| IBIS file stm32mp151_153xad_tfbga257.ibs
[IBIS ver]   4.2
[File name]   stm32mp151_153xad_tfbga257.ibs
[File Rev]   2.2
[Date]   07-07-2026
[Source]   Data Created at STMicroelectronics
[Disclaimer]  This information is for modeling purpose only and is
   not guaranted.
   The information is subject to change without notice.
[Copyright]   Copyright 2026 STMicroelectronics Inc.
|   Component stm32mp151_153xad_tfbga257
[Component] stm32mp151_153xad_tfbga257
[Manufacturer] STMicroelectronics
[Package]
| variable   typ   min   max
R_pkg  4.52E-01  1.78E-01  6.98E-01
L_pkg  2.44E-09  9.38E-10  4.05E-09
C_pkg  6.28E-13  3.36E-13  3.08E-12
[Pin]   signal_name   model_name
1A1  PE1  io8_ft
1A2  PD10  io8_ft_hslv
1A3  PE3  io8_ft_hslv
1A4  PB14  io8_ft_hslv
1A5  PD2  io8_ft_hslv
1A6  VSS  gnd
1A7  VDD1V2_Unused  nc
1A8  DDR_ZQ  nc
1A9  DDR_A7  PDDRIO_PAD
1B1  PD6  io8_ft_hslv
1B2  PE14  io8_ft_hslv
1B3  VDDCORE  power
1B4  PC12  io8_ft_hslv
1B5  VDDCORE  power
1B6  VDDA1V8_Unused  nc
1B7  VDD1V2_Unused  nc
1B8  VSS  gnd
1B9  VDDQ_DDR  power
1C1  PD9  io8_ft
1C2  PD15  io8_ft
1C3  VSS  gnd
1C4  VDDCORE  power
1C5  VSS  gnd
1C6  VDDCORE  power
1C7  VSS  gnd
1C8  DDR_DTO1  PDDRIO_PAD
1C9  DDR_A5  PDDRIO_PAD
1D1  VBAT  power
1D2  VSS  gnd
1D3  VDDCORE  power
1D4  VSS  gnd
1D5  VDDCORE  power
1D6  VSS  gnd
1D7  VDDCORE  power
1D8  DDR_DTO0  PDDRIO_PAD
1D9  VDDQ_DDR  power
1E1  PD14  io8_ft
1E2  VDD  power
1E3  VSS  gnd
1E4  VDDCORE  power
1E5  VSS  gnd
1E6  VDDCORE  power
1E7  VSS  gnd
1E8  VDDCORE  power
1E9  DDR_RASN  PDDRIO_PAD
1F1  VDDA  nc
1F2  VDDA  nc
1F3  VDD  power
1F4  VSS  gnd
1F5  VDDCORE  power
1F6  VSS  gnd
1F7  VDDCORE  power
1F8  DDR_ATO  nc
1F9  VDDQ_DDR  power
1G1  VSSA  gnd
1G2  VSS  gnd
1G3  VDD  power
1G4  VDD  power
1G5  VSS  gnd
1G6  VDDCORE  power
1G7  VSS  gnd
1G8  VDDCORE  power
1G9  DDR_A6  PDDRIO_PAD
1H1  PA5  io8_ft_hslv
1H2  VSS  gnd
1H3  VSS  gnd
1H4  VSS  gnd
1H5  VDDA1V8_REG  nc
1H6  VSS  gnd
1H7  VDD3V3_USB  power
1H8  VSS  gnd
1H9  VDDQ_DDR  power
1J1  PA4  io8_ft
1J2  PB13  io8_ft_hslv_et
1J3  VDD_OTP  power
1J4  PE9  io8_ft_hslv
1J5  VSS  gnd
1J6  VDDA1V1_REG  nc
1J7  PF10  io8_ft_hslv
1J8  USB_RREF  nc
1J9  VSS  gnd
A1  VSS  gnd
A2  PD1  io8_ft_hslv
A3  PB7  io8_ft_hslv
A4  PC6  io8_ft_hslv
A6  VSS  gnd
A7  PD3  io8_ft_hslv
A9  PC8  io8_ft_hslv
A10  PE4  io8_ft_hslv
A12  DNU  nc
A13  DNU  nc
A15  JTDO-TRACESWO  io8_ft
A16  JTCK-SWCLK  isudqf
A17  DDR_DQ0  PDDRIO_PAD
A18  DDR_DQ1  PDDRIO_PAD
A19  VSS  gnd
B1  PG15  io8_ft_hslv
B2  PE6  io8_ft_hslv
B3  PD7  io8_ft_hslv
B4  PA15  io8_ft_hslv
B5  PG6  io8_ft_hslv
B6  PB4  io8_ft_hslv
B7  PE5  io8_ft_hslv
B8  PA8  io8_ft_hslv
B9  PC9  io8_ft_hslv
B10  PC10  io8_ft_hslv
B11  DNU  nc
B12  DNU  nc
B13  DNU  nc
B14  NJTRST  isudqf
B15  JTDI  isudqf
B16  DDR_DQ3  PDDRIO_PAD
B17  DDR_DQ7  PDDRIO_PAD
B18  DDR_DQS0N  PDIFF_PAD
B19  DDR_DQS0P  PDIFF_PAD
C1  PE12  io8_ft_hslv
C2  PE0  io8_ft_hslv
C3  PD4  io8_ft_hslv
C4  PD5  io8_ft_hslv
C5  PD0  io8_ft_hslv
C6  PA9  io8_ft_hslv
C7  PB3  io8_ft_hslv
C8  PB15  io8_ft_hslv
C9  PB9  io8_ft_hslv
C10  PC7  io8_ft_hslv
C11  PC11  io8_ft_hslv
C12  DNU  nc
C13  VDD_Unused  power
C14  VSS  gnd
C15  JTMS-SWDIO  io8_ft
C16  DDR_RESETN  PDDRIO_PAD
C17  DDR_DQM0  PDDRIO_PAD
C18  DDR_DQ2  PDDRIO_PAD
C19  DDR_DQ6  PDDRIO_PAD
D1  PG12  io8_ft_hslv
D2  PE11  io8_ft
D3  PE15  io8_ft
D17  VSS  gnd
D18  DDR_DQ4  PDDRIO_PAD
D19  DDR_DQ5  PDDRIO_PAD
E1  PD8  io8_ft
|E2  NRST  ioreset_ft_v33
E2  NRST  nc
E3  PE13  io8_ft_hslv
E17  DDR_A13  PDDRIO_PAD
E18  DDR_A9  PDDRIO_PAD
F2  PC15-OSC32_OUT  io8_ft
F3  VSS  gnd
F17  DDR_A2  PDDRIO_PAD
F18  VSS  gnd
F19  DDR_A3  PDDRIO_PAD
G1  VSS  gnd
G2  PC14-OSC32_IN  io8_ft
G3  PC13  io8_ft
G17  VSS  gnd
G18  DDR_A0  PDDRIO_PAD
G19  DDR_BA0  PDDRIO_PAD
H1  BOOT2  isudqf
H2  PH0-OSC_IN  io8_ft
H3  BOOT0  isudqf
H17  DDR_BA2  PDDRIO_PAD
H18  DDR_ODT  PDDRIO_PAD
J2  PH1-OSC_OUT  io8_ft
J3  NRST_CORE  isudqf
J17  DDR_CSN  PDDRIO_PAD
J18  DDR_WEN  PDDRIO_PAD
J19  DDR_CASN  PDDRIO_PAD
K1  PWR_LP  io8_ft
K2  PDR_ON_CORE  isudqf
K3  BOOT1  isudqf
K17  VSS  gnd
K18  DDR_CLKN  PDDRIO_PAD
K19  VSS  gnd
L1  PA14  io8_ft
L2  PA13  io8_ft
L3  PDR_ON  isudqf
L17  DDR_CLKP  PDDRIO_PAD
L18  DDR_A15  PDDRIO_PAD
M2  PWR_ON  io8_ft
M3  VREF+  nc
M17  DDR_A10  PDDRIO_PAD
M18  DDR_A12  PDDRIO_PAD
M19  DDR_A1  PDDRIO_PAD
N1  VSS  gnd
N2  PA3  io8_ft
N3  PA0  io8_ft_hslv
N17  VSS  gnd
N18  DDR_A14  PDDRIO_PAD
N19  DDR_A11  PDDRIO_PAD
P1  PE2  io8_ft_et_i2c_hslv
P2  PC2  io8_ft_hslv_et
P3  PC3  io8_ft_hslv
P17  DDR_CKE  PDDRIO_PAD
P18  DDR_BA1  PDDRIO_PAD
R2  PG14  io8_ft_hslv_et
R3  PG13  io8_ft_hslv_et
R17  DDR_A4  PDDRIO_PAD
R18  DDR_DQ8  PDDRIO_PAD
R19  VSS  gnd
T1  PA1  io8_ft_hslv
T2  PC1  io8_ft_hslv
T3  PA2  io8_ft_hslv
T17  DDR_A8  PDDRIO_PAD
T18  DDR_DQ13  PDDRIO_PAD
T19  DDR_DQ10  PDDRIO_PAD
U1  PB1  io8_ft
U2  PB0  io8_ft
U3  PB11  io8_ft_et_i2c_hslv
U4  PC0  io8_ft_hslv
U5  PB10  io8_ft_i2c_hslv
U6  PG11  io8_ft_hslv_et
U7  PG10  io8_ft_hslv
U8  PD11  io8_ft_hslv
U9  VSS  gnd
U10  PF6  io8_ft_hslv
U11  BYPASS_REG1V8  isudqf
U12  PE8  io8_ft_hslv
U13  PD13  io8_ft_i2c_hslv
U14  PD12  io8_ft_i2c_hslv
U15  PA11  io8_i2c_usb_lsfs_bcd_otg20_ft
U16  PA10  io8usb_id_otg20_ft
U17  DDR_DQ14  PDDRIO_PAD
U18  DDR_DQS1N  PDIFF_PAD
U19  DDR_DQ9  PDDRIO_PAD
V1  PC5  io8_ft
V2  PC4  io8_ft
V3  PB12  io8_ft_hslv_et
V4  PB8  io8_ft_et_i2c_hslv
V5  PB5  io8_ft_hslv_et
V6  PG8  io8_ft_hslv_et
V7  PE7  io8_ft_hslv
V8  PF8  io8_ft_hslv
V9  PF9  io8_ft_hslv
V10  USB_DP2  nc
V11  PG7  io8_ft_hslv
V12  PE10  io8_ft_hslv
V13  PB2  io8_ft_hslv
V14  USB_DP1  nc
V15  PA12  io8_i2c_usb_lsfs_bcd_otg20_ft
V16  OTG_VBUS  io8usb_vbus_otg20_ft
V17  DDR_DQ15  PDDRIO_PAD
V18  DDR_DM1  PDDRIO_PAD
V19  DDR_DQS1P  PDIFF_PAD
W1  VSS  gnd
W2  PA7  io8_ft_hslv
W3  PA6  io8_ft_hslv
W4  PF11  io8_ft_hslv
W5  VSS  gnd
W7  PF7  io8_ft_hslv
W8  PG9  io8_ft_hslv
W10  USB_DM2  nc
W11  PB6  io8_ft_i2c_hslv
W13  VSS  gnd
W14  USB_DM1  nc
W16  DDR_VREF  POWER
W17  DDR_DQ12  PDDRIO_PAD
W18  DDR_DQ11  PDDRIO_PAD
W19  VSS  gnd
[Package Model]   500-tfbga-10x10-257-100mhz-181019
[Pin Mapping]   pulldown_ref   pullup_ref   | Comment
1A1  VSS  VDD
1A2  VSS  VDD
1A3  VSS  VDD
1A4  VSS  VDD
1A5  VSS  VDD
1A6  VSS  nc
1A7  nc  nc
1A8  nc nc
1A9  VSS  VDDQ_DDR
1B1  VSS  VDD
1B2  VSS  VDD
1B3  nc  VDDCORE
1B4  VSS  VDD
1B5  nc  VDDCORE
1B6  nc  nc
1B7  nc  nc
1B8  VSS  nc
1B9  nc  VDDQ_DDR
1C1  VSS  VDD
1C2  VSS  VDD
1C3  VSS  nc
1C4  nc  VDDCORE
1C5  VSS  nc
1C6  nc  VDDCORE
1C7  VSS  nc
1C8  VSS  VDDQ_DDR
1C9  VSS  VDDQ_DDR
1D1  nc  VDD_sw
1D2  VSS  nc
1D3  nc  VDDCORE
1D4  VSS  nc
1D5  nc  VDDCORE
1D6  VSS  nc
1D7  nc  VDDCORE
1D8  VSS  VDDQ_DDR
1D9  nc  VDDQ_DDR
1E1  VSS  VDD
1E2  nc  VDD
1E3  VSS  nc
1E4  nc  VDDCORE
1E5  VSS  nc
1E6  nc  VDDCORE
1E7  VSS  nc
1E8  nc  VDDCORE
1E9  VSS  VDDQ_DDR
1F1  nc  nc
1F2  nc  nc
1F3  nc  VDD
1F4  VSS  nc
1F5  nc  VDDCORE
1F6  VSS  nc
1F7  nc  VDDCORE
1F8  nc  nc
1F9  nc  VDDQ_DDR
1G1  VSS  nc
1G2  VSS  nc
1G3  nc  VDD
1G4  nc  VDD
1G5  VSS  nc
1G6  nc  VDDCORE
1G7  VSS  nc
1G8  nc  VDDCORE
1G9  VSS  VDDQ_DDR
1H1  VSS  VDD
1H2  VSS  nc
1H3  VSS  nc
1H4  VSS  nc
1H5  nc  nc
1H6  VSS  nc
1H7  nc  VDD3V3_USB
1H8  VSS  nc
1H9  nc  VDDQ_DDR
1J1  VSS  VDD
1J2  VSS  VDD
1J3  nc  VDD
1J4  VSS  VDD
1J5  VSS  nc
1J6  nc  nc
1J7  VSS  VDD
1J8  nc nc
1J9  VSS  nc
A1  VSS  nc
A2  VSS  VDD
A3  VSS  VDD
A4  VSS  VDD
A6  VSS  nc
A7  VSS  VDD
A9  VSS  VDD
A10  VSS  VDD
A12  nc nc
A13  nc nc
A15  VSS  VDD
A16  VSS  VDD
A17  VSS  VDDQ_DDR
A18  VSS  VDDQ_DDR
A19  VSS  nc
B1  VSS  VDD
B2  VSS  VDD
B3  VSS  VDD
B4  VSS  VDD
B5  VSS  VDD
B6  VSS  VDD
B7  VSS  VDD
B8  VSS  VDD
B9  VSS  VDD
B10  VSS  VDD
B11  nc nc
B12  nc nc
B13  nc nc
B14  VSS  VDD
B15  VSS  VDD
B16  VSS  VDDQ_DDR
B17  VSS  VDDQ_DDR
B18  VSS  VDDQ_DDR
B19  VSS  VDDQ_DDR
C1  VSS  VDD
C2  VSS  VDD
C3  VSS  VDD
C4  VSS  VDD
C5  VSS  VDD
C6  VSS  VDD
C7  VSS  VDD
C8  VSS  VDD
C9  VSS  VDD
C10  VSS  VDD
C11  VSS  VDD
C12  nc nc
C13  nc  vdd_Unused
C14  VSS  nc
C15  VSS  VDD
C16  VSS  VDDQ_DDR
C17  VSS  VDDQ_DDR
C18  VSS  VDDQ_DDR
C19  VSS  VDDQ_DDR
D1  VSS  VDD
D2  VSS  VDD
D3  VSS  VDD
D17  VSS  nc
D18  VSS  VDDQ_DDR
D19  VSS  VDDQ_DDR
E1  VSS  VDD
E2  nc  nc
E3  VSS  VDD
E17  VSS  VDDQ_DDR
E18  VSS  VDDQ_DDR
F2  nc  nc
F3  VSS  nc
F17  VSS  VDDQ_DDR
F18  VSS  nc
F19  VSS  VDDQ_DDR
G1  VSS  nc
G2  nc  nc
G3  nc  nc
G17  VSS  nc
G18  VSS  VDDQ_DDR
G19  VSS  VDDQ_DDR
H1  VSS  VDD
H2  VSS  VDD
H3  VSS  VDD
H17  VSS  VDDQ_DDR
H18  VSS  VDDQ_DDR
J2  VSS  VDD
J3  VSS  VDD
J17  VSS  VDDQ_DDR
J18  VSS  VDDQ_DDR
J19  VSS  VDDQ_DDR
K1  VSS  VDD
K2  VSS  VDD
K3  VSS  VDD
K17  VSS  nc
K18  VSS  VDDQ_DDR
K19  VSS  nc
L1  VSS  VDD
L2  VSS  VDD
L3  VSS  VDD
L17  VSS  VDDQ_DDR
L18  VSS  VDDQ_DDR
M2  VSS  VDD
M3  nc  nc
M17  VSS  VDDQ_DDR
M18  VSS  VDDQ_DDR
M19  VSS  VDDQ_DDR
N1  VSS  nc
N2  VSS  VDD
N3  VSS  VDD
N17  VSS  nc
N18  VSS  VDDQ_DDR
N19  VSS  VDDQ_DDR
P1  VSS  VDD
P2  VSS  VDD
P3  VSS  VDD
P17  VSS  VDDQ_DDR
P18  VSS  VDDQ_DDR
R2  VSS  VDD
R3  VSS  VDD
R17  VSS  VDDQ_DDR
R18  VSS  VDDQ_DDR
R19  VSS  nc
T1  VSS  VDD
T2  VSS  VDD
T3  VSS  VDD
T17  VSS  VDDQ_DDR
T18  VSS  VDDQ_DDR
T19  VSS  VDDQ_DDR
U1  VSS  VDD
U2  VSS  VDD
U3  VSS  VDD
U4  VSS  VDD
U5  VSS  VDD
U6  VSS  VDD
U7  VSS  VDD
U8  VSS  VDD
U9  VSS  nc
U10  VSS  VDD
U11  VSS  VDD
U12  VSS  VDD
U13  VSS  VDD
U14  VSS  VDD
U15  VSS  VDD3V3_USB  | Depending on IO usage
| U15  VSS  VDD  | Depending on IO usage
U16  VSS  VDD3V3_USB  | Depending on IO usage
| U16  VSS  VDD  | Depending on IO usage
U17  VSS  VDDQ_DDR
U18  VSS  VDDQ_DDR
U19  VSS  VDDQ_DDR
V1  VSS  VDD
V2  VSS  VDD
V3  VSS  VDD
V4  VSS  VDD
V5  VSS  VDD
V6  VSS  VDD
V7  VSS  VDD
V8  VSS  VDD
V9  VSS  VDD
V10  nc nc
V11  VSS  VDD
V12  VSS  VDD
V13  VSS  VDD
V14  nc nc
V15  VSS  VDD3V3_USB  | Depending on IO usage
| V15  VSS  VDD  | Depending on IO usage
V16  VSS  VDD3V3_USB  | Depending on IO usage
| V16  VSS  VDD  | Depending on IO usage
V17  VSS  VDDQ_DDR
V18  VSS  VDDQ_DDR
V19  VSS  VDDQ_DDR
W1  VSS  nc
W2  VSS  VDD
W3  VSS  VDD
W4  VSS  VDD
W5  VSS  nc
W7  VSS  VDD
W8  VSS  VDD
W10  nc nc
W11  VSS  VDD
W13  VSS  nc
W14  nc nc
W16  nc  VDDQ_DDR
W17  VSS  VDDQ_DDR
W18  VSS  VDDQ_DDR
W19  VSS  nc
|**********************DIFF PIN*********************************************
[Diff_pin]   inv_pin   vdiff   tdelay_typ   tdelay_min   tdelay_max
   L17   K18   0.320V   0ns   NA   NA   |CK
   B18   B19   0.320V   0ns   NA   NA   |DQS0
   U18   V19   0.320V   0ns   NA   NA   |DQS1
[Model Selector] io8usb_id_otg20_ft
io8_ft_ls_1v2   "GPIO - 5V tolerant - 1.2V range - Low speed"
io8_ft_ms_1v2   "GPIO - 5V tolerant - 1.2V range - Med speed"
io8_ft_hs_1v2   "GPIO - 5V tolerant - 1.2V range - High speed"
io8_ft_fs_1v2   "GPIO - 5V tolerant - 1.2V range - Fast speed"
io8_ft_hs_1v8   "GPIO - 5V tolerant - 1.8V range - High speed"
io8_ft_fs_1v8   "GPIO - 5V tolerant - 1.8V range - Fast speed"
io8_ft_ms_1v8   "GPIO - 5V tolerant - 1.8V range - Med speed"
io8_ft_ls_1v8   "GPIO - 5V tolerant - 1.8V range - Low speed"
io8_ft_hs_3v3   "GPIO - 5V tolerant - 3.3V range - High speed"
io8_ft_fs_3v3   "GPIO - 5V tolerant - 3.3V range - Fast speed"
io8_ft_ms_3v3   "GPIO - 5V tolerant - 3.3V range - Med speed"
io8_ft_ls_3v3   "GPIO - 5V tolerant - 3.3V range - Low speed"
[Model Selector] io8usb_vbus_otg20_ft
io8_ft_ls_1v2   "GPIO - 5V tolerant - 1.2V range - Low speed"
io8_ft_ms_1v2   "GPIO - 5V tolerant - 1.2V range - Med speed"
io8_ft_hs_1v2   "GPIO - 5V tolerant - 1.2V range - High speed"
io8_ft_fs_1v2   "GPIO - 5V tolerant - 1.2V range - Fast speed"
io8_ft_hs_1v8   "GPIO - 5V tolerant - 1.8V range - High speed"
io8_ft_fs_1v8   "GPIO - 5V tolerant - 1.8V range - Fast speed"
io8_ft_ms_1v8   "GPIO - 5V tolerant - 1.8V range - Med speed"
io8_ft_ls_1v8   "GPIO - 5V tolerant - 1.8V range - Low speed"
io8_ft_hs_3v3   "GPIO - 5V tolerant - 3.3V range - High speed"
io8_ft_fs_3v3   "GPIO - 5V tolerant - 3.3V range - Fast speed"
io8_ft_ms_3v3   "GPIO - 5V tolerant - 3.3V range - Med speed"
io8_ft_ls_3v3   "GPIO - 5V tolerant - 3.3V range - Low speed"
[Model Selector] io8_ft
io8_ft_ls_1v2   "GPIO - 5V tolerant - 1.2V range - Low speed"
io8_ft_ms_1v2   "GPIO - 5V tolerant - 1.2V range - Med speed"
io8_ft_hs_1v2   "GPIO - 5V tolerant - 1.2V range - High speed"
io8_ft_fs_1v2   "GPIO - 5V tolerant - 1.2V range - Fast speed"
io8_ft_hs_1v8   "GPIO - 5V tolerant - 1.8V range - High speed"
io8_ft_fs_1v8   "GPIO - 5V tolerant - 1.8V range - Fast speed"
io8_ft_ms_1v8   "GPIO - 5V tolerant - 1.8V range - Med speed"
io8_ft_ls_1v8   "GPIO - 5V tolerant - 1.8V range - Low speed"
io8_ft_hs_3v3   "GPIO - 5V tolerant - 3.3V range - High speed"
io8_ft_fs_3v3   "GPIO - 5V tolerant - 3.3V range - Fast speed"
io8_ft_ms_3v3   "GPIO - 5V tolerant - 3.3V range - Med speed"
io8_ft_ls_3v3   "GPIO - 5V tolerant - 3.3V range - Low speed"
[Model Selector] io8_ft_hslv
io8_ft_ls_1v2   "GPIO - 5V tolerant - 1.2V range - Low speed"
io8_ft_ms_1v2   "GPIO - 5V tolerant - 1.2V range - Med speed"
io8_ft_hs_1v2   "GPIO - 5V tolerant - 1.2V range - High speed"
io8_ft_fs_1v2   "GPIO - 5V tolerant - 1.2V range - Fast speed"
io8_ft_hs_1v8   "GPIO - 5V tolerant - 1.8V range - High speed"
io8_ft_fs_1v8   "GPIO - 5V tolerant - 1.8V range - Fast speed"
io8_ft_ms_1v8   "GPIO - 5V tolerant - 1.8V range - Med speed"
io8_ft_ls_1v8   "GPIO - 5V tolerant - 1.8V range - Low speed"
io8_ft_hs_3v3   "GPIO - 5V tolerant - 3.3V range - High speed"
io8_ft_fs_3v3   "GPIO - 5V tolerant - 3.3V range - Fast speed"
io8_ft_ms_3v3   "GPIO - 5V tolerant - 3.3V range - Med speed"
io8_ft_ls_3v3   "GPIO - 5V tolerant - 3.3V range - Low speed"
io8_ft_hslv_hs_1v2   "GPIO - hslv opt - 5V tolerant - 1.2V range - High speed"
io8_ft_hslv_fs_1v2   "GPIO - hslv opt - 5V tolerant - 1.2V range - Fast speed"
io8_ft_hslv_ms_1v2   "GPIO - hslv opt - 5V tolerant - 1.2V range - Med speed"
io8_ft_hslv_ls_1v2   "GPIO - hslv opt - 5V tolerant - 1.2V range - Low speed"
io8_ft_hslv_hs_1v8   "GPIO - hslv opt - 5V tolerant - 1.8V range - High speed"
io8_ft_hslv_fs_1v8   "GPIO - hslv opt - 5V tolerant - 1.8V range - Fast speed"
io8_ft_hslv_ms_1v8   "GPIO - hslv opt - 5V tolerant - 1.8V range - Med speed"
io8_ft_hslv_ls_1v8   "GPIO - hslv opt - 5V tolerant - 1.8V range - Low speed"
io8_ft_hslv_hs_2v5   "GPIO - hslv opt - 5V tolerant - 2.5V range - High speed"
io8_ft_hslv_fs_2v5   "GPIO - hslv opt - 5V tolerant - 2.5V range - Fast speed"
io8_ft_hslv_ms_2v5   "GPIO - hslv opt - 5V tolerant - 2.5V range - Med speed"
io8_ft_hslv_ls_2v5   "GPIO - hslv opt - 5V tolerant - 2.5V range - Low speed"
[Model Selector] io8_ft_hslv_et
io8_ft_et_ls_1v2   "GPIO - Ethernet - 5V tol - 1.2V range - Low speed"
io8_ft_et_ms_1v2   "GPIO - Ethernet - 5V tol - 1.2V range - Med speed"
io8_ft_et_hs_1v2   "GPIO - Ethernet - 5V tol - 1.2V range - High speed"
io8_ft_et_fs_1v2   "GPIO - Ethernet - 5V tol - 1.2V range - Fast speed"
io8_ft_et_hs_1v8   "GPIO - Ethernet - 5V tol - 1.8V range - High speed"
io8_ft_et_fs_1v8   "GPIO - Ethernet - 5V tol - 1.8V range - Fast speed"
io8_ft_et_ms_1v8   "GPIO - Ethernet - 5V tol - 1.8V range - Med speed"
io8_ft_et_ls_1v8   "GPIO - Ethernet - 5V tol - 1.8V range - Low speed"
io8_ft_et_hs_3v3   "GPIO - Ethernet - 5V tol - 3.3V range - High speed"
io8_ft_et_fs_3v3   "GPIO - Ethernet - 5V tol - 3.3V range - Fast speed"
io8_ft_et_ms_3v3   "GPIO - Ethernet - 5V tol - 3.3V range - Med speed"
io8_ft_et_ls_3v3   "GPIO - Ethernet - 5V tol - 3.3V range - Low speed"
io8_ft_et_hslv_ls_1v2   "GPIO - hslv opt - Ethernet - 5V tol - 1.2V range - Low speed"
io8_ft_et_hslv_hs_1v2   "GPIO - hslv opt - Ethernet - 5V tol - 1.2V range - High speed"
io8_ft_et_hslv_fs_1v2   "GPIO - hslv opt - Ethernet - 5V tol - 1.2V range - Fast speed"
io8_ft_et_hslv_ms_1v2   "GPIO - hslv opt - Ethernet - 5V tol - 1.2V range - Med speed"
io8_ft_et_hslv_ls_1v8   "GPIO - hslv opt - Ethernet - 5V tol - 1.8V range - Low speed"
io8_ft_et_hslv_hs_1v8   "GPIO - hslv opt - Ethernet - 5V tol - 1.8V range - High speed"
io8_ft_et_hslv_fs_1v8   "GPIO - hslv opt - Ethernet - 5V tol - 1.2V range - Fast speed"
io8_ft_et_hslv_ms_1v8   "GPIO - hslv opt - Ethernet - 5V tol - 1.8V range - Med speed"
io8_ft_et_hslv_hs_2v5   "GPIO - hslv opt - Ethernet - 5V tol - 2.5V range - High speed"
io8_ft_et_hslv_fs_2v5   "GPIO - hslv opt - Ethernet - 5V tol - 2.5V range - Fast speed"
io8_ft_et_hslv_ms_2v5   "GPIO - hslv opt - Ethernet - 5V tol - 2.5V range - Med speed"
io8_ft_et_hslv_ls_2v5   "GPIO - hslv opt - Ethernet - 5V tol - 2.5V range - Low speed"
[Model Selector] io8_ft_et_i2c_hslv
io8_ft_et_ls_1v2   "GPIO - 5V tol - 1.2V range - Low speed"
io8_ft_et_ms_1v2   "GPIO - 5V tol - 1.2V range - Med speed"
io8_ft_et_hs_1v2   "GPIO - 5V tol - 1.2V range - High speed"
io8_ft_et_fs_1v2   "GPIO - 5V tol - 1.2V range - Fast speed"
io8_ft_et_hs_1v8   "GPIO - 5V tol - 1.8V range - High speed"
io8_ft_et_fs_1v8   "GPIO - 5V tol - 1.8V range - Fast speed"
io8_ft_et_ms_1v8   "GPIO - 5V tol - 1.8V range - Med speed"
io8_ft_et_ls_1v8   "GPIO - 5V tol - 1.8V range - Low speed"
io8_ft_et_hs_3v3   "GPIO - 5V tol - 3.3V range - High speed"
io8_ft_et_fs_3v3   "GPIO - 5V tol - 3.3V range - Fast speed"
io8_ft_et_ms_3v3   "GPIO - 5V tol - 3.3V range - Med speed"
io8_ft_et_ls_3v3   "GPIO - 5V tol - 3.3V range - Low speed"
io8_ft_et_hslv_ls_1v2   "GPIO - hslv opt -Ethernet - 5V tol - 1.2V range - Low speed"
io8_ft_et_hslv_hs_1v2   "GPIO - hslv opt -Ethernet - 5V tol - 1.2V range - High speed"
io8_ft_et_hslv_fs_1v2   "GPIO - hslv opt -Ethernet - 5V tol - 1.2V range - Fast speed"
io8_ft_et_hslv_ms_1v2   "GPIO - hslv opt -Ethernet - 5V tol - 1.2V range - Med speed"
io8_ft_et_hslv_ls_1v8   "GPIO - hslv opt -Ethernet - 5V tol - 1.8V range - Low speed"
io8_ft_et_hslv_hs_1v8   "GPIO - hslv opt -Ethernet - 5V tol - 1.8V range - High speed"
io8_ft_et_hslv_fs_1v8   "GPIO - hslv opt -Ethernet - 5V tol - 1.2V range - Fast speed"
io8_ft_et_hslv_ms_1v8   "GPIO - hslv opt -Ethernet - 5V tol - 1.8V range - Med speed"
io8_ft_et_hslv_hs_2v5   "GPIO - hslv opt -Ethernet - 5V tol - 2.5V range - High speed"
io8_ft_et_hslv_fs_2v5   "GPIO - hslv opt  -Ethernet- 5V tol - 2.5V range - Fast speed"
io8_ft_et_hslv_ms_2v5   "GPIO - hslv opt -Ethernet - 5V tol - 2.5V range - Med speed"
io8_ft_et_hslv_ls_2v5   "GPIO - hslv opt -Ethernet - 5V tol - 2.5V range - Low speed"
io8_ft_i2c_1v2   "GPIO - 5V tolerant - 1.2V range - Open drain"
io8_ft_i2c_1v8   "GPIO - 5V tolerant - 1.8V range - Open drain"
io8_ft_i2c_3v3   "GPIO - 5V tolerant - 3.3V range - Open drain"
io8_ft_i2c_hslv_1v2   "GPIO - hslv opt - 5V tolerant - 1.2V range - Open drain"
io8_ft_i2c_hslv_1v8   "GPIO - hslv opt - 5V tolerant - 1.8V range - Open drain"
io8_ft_i2c_hslv_2v5   "GPIO - hslv opt - 5V tolerant - 2.5V range - Open drain"
[Model Selector] io8_ft_i2c_hslv
io8_ft_ls_1v2   "GPIO - 5V tolerant - 1.2V range - Low speed"
io8_ft_ms_1v2   "GPIO - 5V tolerant - 1.2V range - Med speed"
io8_ft_hs_1v2   "GPIO - 5V tolerant - 1.2V range - High speed"
io8_ft_fs_1v2   "GPIO - 5V tolerant - 1.2V range - Fast speed"
io8_ft_hs_1v8   "GPIO - 5V tolerant - 1.8V range - High speed"
io8_ft_fs_1v8   "GPIO - 5V tolerant - 1.8V range - Fast speed"
io8_ft_ms_1v8   "GPIO - 5V tolerant - 1.8V range - Med speed"
io8_ft_ls_1v8   "GPIO - 5V tolerant - 1.8V range - Low speed"
io8_ft_hs_3v3   "GPIO - 5V tolerant - 3.3V range - High speed"
io8_ft_fs_3v3   "GPIO - 5V tolerant - 3.3V range - Fast speed"
io8_ft_ms_3v3   "GPIO - 5V tolerant - 3.3V range - Med speed"
io8_ft_ls_3v3   "GPIO - 5V tolerant - 3.3V range - Low speed"
io8_ft_hslv_hs_1v2   "GPIO - hslv opt - 5V tolerant - 1.2V range - High speed"
io8_ft_hslv_fs_1v2   "GPIO - hslv opt - 5V tolerant - 1.2V range - Fast speed"
io8_ft_hslv_ms_1v2   "GPIO - hslv opt - 5V tolerant - 1.2V range - Med speed"
io8_ft_hslv_ls_1v2   "GPIO - hslv opt - 5V tolerant - 1.2V range - Low speed"
io8_ft_hslv_hs_1v8   "GPIO - hslv opt - 5V tolerant - 1.8V range - High speed"
io8_ft_hslv_fs_1v8   "GPIO - hslv opt - 5V tolerant - 1.8V range - Fast speed"
io8_ft_hslv_ms_1v8   "GPIO - hslv opt - 5V tolerant - 1.8V range - Med speed"
io8_ft_hslv_ls_1v8   "GPIO - hslv opt - 5V tolerant - 1.8V range - Low speed"
io8_ft_hslv_hs_2v5   "GPIO - hslv opt - 5V tolerant - 2.5V range - High speed"
io8_ft_hslv_fs_2v5   "GPIO - hslv opt - 5V tolerant - 2.5V range - Fast speed"
io8_ft_hslv_ms_2v5   "GPIO - hslv opt - 5V tolerant - 2.5V range - Med speed"
io8_ft_hslv_ls_2v5   "GPIO - hslv opt - 5V tolerant - 2.5V range - Low speed"
io8_ft_i2c_1v2   "GPIO - 5V tolerant - 1.2V range - Open drain"
io8_ft_i2c_1v8   "GPIO - 5V tolerant - 1.8V range - Open drain"
io8_ft_i2c_3v3   "GPIO - 5V tolerant - 3.3V range - Open drain"
io8_ft_i2c_hslv_1v2   "GPIO - hslv opt - 5V tolerant - 1.2V range - Open drain"
io8_ft_i2c_hslv_1v8   "GPIO - hslv opt - 5V tolerant - 1.8V range - Open drain"
io8_ft_i2c_hslv_2v5   "GPIO - hslv opt - 5V tolerant - 2.5V range - Open drain"
[Model Selector] io8_i2c_usb_lsfs_bcd_otg20_ft
io8_ft_ls_1v2   "GPIO - 5V tolerant - 1.2V range - Low speed"
io8_ft_ms_1v2   "GPIO - 5V tolerant - 1.2V range - Med speed"
io8_ft_hs_1v2   "GPIO - 5V tolerant - 1.2V range - High speed"
io8_ft_fs_1v2   "GPIO - 5V tolerant - 1.2V range - Fast speed"
io8_ft_hs_1v8   "GPIO - 5V tolerant - 1.8V range - High speed"
io8_ft_fs_1v8   "GPIO - 5V tolerant - 1.8V range - Fast speed"
io8_ft_ms_1v8   "GPIO - 5V tolerant - 1.8V range - Med speed"
io8_ft_ls_1v8   "GPIO - 5V tolerant - 1.8V range - Low speed"
io8_ft_hs_3v3   "GPIO - 5V tolerant - 3.3V range - High speed"
io8_ft_fs_3v3   "GPIO - 5V tolerant - 3.3V range - Fast speed"
io8_ft_ms_3v3   "GPIO - 5V tolerant - 3.3V range - Med speed"
io8_ft_ls_3v3   "GPIO - 5V tolerant - 3.3V range - Low speed"
io8_ft_i2c_1v2   "GPIO - 5V tolerant - 1.2V range - Open drain"
io8_ft_i2c_1v8   "GPIO - 5V tolerant - 1.8V range - Open drain"
io8_ft_i2c_3v3   "GPIO - 5V tolerant - 3.3V range - Open drain"
io8usb_ft_hs_3v3   "USB full speed"
io8usb_ft_ls_3v3   "USB low speed"
|[Model Selector] ioreset_ft_v33
|ioreset_ft_v33_1v2   "Reset PAD. 5V tolerant. 1.2V range"
|ioreset_ft_v33_1v8   "Reset PAD. 5V tolerant. 1.8V range"
|ioreset_ft_v33_3v3   "Reset PAD. 5V tolerant. 3.3V range"
[Model Selector] isudqf
isudqf_ft_1v2   "Input Buffer - 5V tolerant - 1.2V range"
isudqf_ft_1v8   "Input Buffer - 5V tolerant - 1.8V range"
isudqf_ft_3v3   "Input Buffer - 5V tolerant - 3.3V range"
[Model Selector] PDIFF_PAD
MSD_D3RF2_18   DDR2 MSD_D3R_PDIFF Z0=18-Ohm
MSD_D3RF2_40   DDR2 MSD_D3R_PDIFF Z0=40-Ohm
MSD_D3RF2_48   DDR2 MSD_D3R_PDIFF Z0=48-Ohm
MSD_D3RF2_ODT150   DDR2 MSD_D3R_PDIFF cell 150-Ohm ODT Receiver
MSD_D3RF2_ODT50   DDR2 MSD_D3R_PDIFF cell 50-Ohm ODT Receiver
MSD_D3RF2_ODT75   DDR2 MSD_D3R_PDIFF cell 75-Ohm ODT Receiver
MSD_D3RF2_ODTOFF   DDR2 MSD_D3R_PDIFF cell ODT off Receiver
MSD_D3RF3_34   DDR3 MSD_D3R_PDIFF cell  Z0=34-Ohm
MSD_D3RF3_40   DDR3 MSD_D3R_PDIFF cell  Z0=40-Ohm
MSD_D3RF3_48   DDR3 MSD_D3R_PDIFF cell  Z0=48-Ohm
MSD_D3RF3L_34   DDR3L MSD_D3R_PDIFF cell  Z0=34-Ohm
MSD_D3RF3L_40   DDR3L MSD_D3R_PDIFF cell  Z0=40-Ohm
MSD_D3RF3L_48   DDR3L MSD_D3R_PDIFF cell  Z0=48-Ohm
MSD_D3RF3L_ODT120   DDR3L MSD_D3R_PDIFF cell 120-Ohm ODT Receiver
MSD_D3RF3L_ODT40   DDR3L MSD_D3R_PDIFF cell 40-Ohm ODT Receiver
MSD_D3RF3L_ODT60   DDR3L MSD_D3R_PDIFF cell 60-Ohm ODT Receiver
MSD_D3RF3L_ODTOFF   DDR3L MSD_D3R_PDIFF cell ODT off Receiver
MSD_D3RF3_ODT120   DDR3 MSD_D3R_PDIFF cell 120-Ohm ODT Receiver
MSD_D3RF3_ODT40   DDR3 MSD_D3R_PDIFF cell 40-Ohm ODT Receiver
MSD_D3RF3_ODT60   DDR3 MSD_D3R_PDIFF cell 60-Ohm ODT Receiver
MSD_D3RF3_ODTOFF   DDR3 MSD_D3R_PDIFF cell ODT off Receiver
MSD_D3RFL2_34   LPDDR2 MSD_D3R_PDIFF cell  Z0=34-Ohm
MSD_D3RFL2_40   LPDDR2 MSD_D3R_PDIFF cell  Z0=40-Ohm
MSD_D3RFL2_48   LPDDR2 MSD_D3R_PDIFF cell  Z0=48-Ohm
MSD_D3RFL2_60   LPDDR2 MSD_D3R_PDIFF cell  Z0=60-Ohm
MSD_D3RFL2_80   LPDDR2 MSD_D3R_PDIFF cell  Z0=80-Ohm
MSD_D3RFL2_ODTOFF   LPDDR2 MSD_D3R_PDIFF cell ODT off Receiver
MSD_D3RFL_48   LPDDR MSD_D3R_PDIFF cell  Z0=48-Ohm
MSD_D3RFL_ODTOFF   LPDDR MSD_D3R_PDIFF cell ODT off Receiver
MSD_D3RF2_18_OPEN   DDR2 MSD_D3R_PDIFF_PDQSR Z0=18-Ohm
MSD_D3RF2_40_OPEN   DDR2 MSD_D3R_PDIFF_PDQSR Z0=40-Ohm
MSD_D3RF2_48_OPEN   DDR2 MSD_D3R_PDIFF_PDQSR Z0=48-Ohm
MSD_D3RF2_18_PD344   DDR2 MSD_D3R_PDIFF_PDQSR Z0=18-Ohm
MSD_D3RF2_40_PD344   DDR2 MSD_D3R_PDIFF_PDQSR Z0=40-Ohm
MSD_D3RF2_48_PD344   DDR2 MSD_D3R_PDIFF_PDQSR Z0=48-Ohm
MSD_D3RF2_18_PD393   DDR2 MSD_D3R_PDIFF_PDQSR Z0=18-Ohm
MSD_D3RF2_40_PD393   DDR2 MSD_D3R_PDIFF_PDQSR Z0=40-Ohm
MSD_D3RF2_48_PD393   DDR2 MSD_D3R_PDIFF_PDQSR Z0=48-Ohm
MSD_D3RF2_18_PD458   DDR2 MSD_D3R_PDIFF_PDQSR Z0=18-Ohm
MSD_D3RF2_40_PD458   DDR2 MSD_D3R_PDIFF_PDQSR Z0=40-Ohm
MSD_D3RF2_48_PD458   DDR2 MSD_D3R_PDIFF_PDQSR Z0=48-Ohm
MSD_D3RF2_18_PD500   DDR2 MSD_D3R_PDIFF_PDQSR Z0=18-Ohm
MSD_D3RF2_40_PD500   DDR2 MSD_D3R_PDIFF_PDQSR Z0=40-Ohm
MSD_D3RF2_48_PD500   DDR2 MSD_D3R_PDIFF_PDQSR Z0=48-Ohm
MSD_D3RF2_18_PD550   DDR2 MSD_D3R_PDIFF_PDQSR Z0=18-Ohm
MSD_D3RF2_40_PD550   DDR2 MSD_D3R_PDIFF_PDQSR Z0=40-Ohm
MSD_D3RF2_48_PD550   DDR2 MSD_D3R_PDIFF_PDQSR Z0=48-Ohm
MSD_D3RF2_18_PD611   DDR2 MSD_D3R_PDIFF_PDQSR Z0=18-Ohm
MSD_D3RF2_40_PD611   DDR2 MSD_D3R_PDIFF_PDQSR Z0=40-Ohm
MSD_D3RF2_48_PD611   DDR2 MSD_D3R_PDIFF_PDQSR Z0=48-Ohm
MSD_D3RF2_18_PD688   DDR2 MSD_D3R_PDIFF_PDQSR Z0=18-Ohm
MSD_D3RF2_40_PD688   DDR2 MSD_D3R_PDIFF_PDQSR Z0=40-Ohm
MSD_D3RF2_48_PD688   DDR2 MSD_D3R_PDIFF_PDQSR Z0=48-Ohm
MSD_D3RF2_18_PU344   DDR2 MSD_D3R_PDIFF_PDQSR Z0=18-Ohm
MSD_D3RF2_40_PU344   DDR2 MSD_D3R_PDIFF_PDQSR Z0=40-Ohm
MSD_D3RF2_48_PU344   DDR2 MSD_D3R_PDIFF_PDQSR Z0=48-Ohm
MSD_D3RF2_18_PU393   DDR2 MSD_D3R_PDIFF_PDQSR Z0=18-Ohm
MSD_D3RF2_40_PU393   DDR2 MSD_D3R_PDIFF_PDQSR Z0=40-Ohm
MSD_D3RF2_48_PU393   DDR2 MSD_D3R_PDIFF_PDQSR Z0=48-Ohm
MSD_D3RF2_18_PU458   DDR2 MSD_D3R_PDIFF_PDQSR Z0=18-Ohm
MSD_D3RF2_40_PU458   DDR2 MSD_D3R_PDIFF_PDQSR Z0=40-Ohm
MSD_D3RF2_48_PU458   DDR2 MSD_D3R_PDIFF_PDQSR Z0=48-Ohm
MSD_D3RF2_18_PU500   DDR2 MSD_D3R_PDIFF_PDQSR Z0=18-Ohm
MSD_D3RF2_40_PU500   DDR2 MSD_D3R_PDIFF_PDQSR Z0=40-Ohm
MSD_D3RF2_48_PU500   DDR2 MSD_D3R_PDIFF_PDQSR Z0=48-Ohm
MSD_D3RF2_18_PU550   DDR2 MSD_D3R_PDIFF_PDQSR Z0=18-Ohm
MSD_D3RF2_40_PU550   DDR2 MSD_D3R_PDIFF_PDQSR Z0=40-Ohm
MSD_D3RF2_48_PU550   DDR2 MSD_D3R_PDIFF_PDQSR Z0=48-Ohm
MSD_D3RF2_18_PU611   DDR2 MSD_D3R_PDIFF_PDQSR Z0=18-Ohm
MSD_D3RF2_40_PU611   DDR2 MSD_D3R_PDIFF_PDQSR Z0=40-Ohm
MSD_D3RF2_48_PU611   DDR2 MSD_D3R_PDIFF_PDQSR Z0=48-Ohm
MSD_D3RF2_18_PU688   DDR2 MSD_D3R_PDIFF_PDQSR Z0=18-Ohm
MSD_D3RF2_40_PU688   DDR2 MSD_D3R_PDIFF_PDQSR Z0=40-Ohm
MSD_D3RF2_48_PU688   DDR2 MSD_D3R_PDIFF_PDQSR Z0=48-Ohm
MSD_D3RF2_18_PWRDWN   DDR2 MSD_D3R_PDIFF_PDQSR Z0=18-Ohm
MSD_D3RF2_40_PWRDWN   DDR2 MSD_D3R_PDIFF_PDQSR Z0=40-Ohm
MSD_D3RF2_48_PWRDWN   DDR2 MSD_D3R_PDIFF_PDQSR Z0=48-Ohm
MSD_D3RF3_34_OPEN   DDR3 MSD_D3R_PDIFF_PDQSR cell  Z0=34-Ohm
MSD_D3RF3_40_OPEN   DDR3 MSD_D3R_PDIFF_PDQSR cell  Z0=40-Ohm
MSD_D3RF3_48_OPEN   DDR3 MSD_D3R_PDIFF_PDQSR cell  Z0=48-Ohm
MSD_D3RF3_34_PD344   DDR3 MSD_D3R_PDIFF_PDQSR cell  Z0=34-Ohm
MSD_D3RF3_40_PD344   DDR3 MSD_D3R_PDIFF_PDQSR cell  Z0=40-Ohm
MSD_D3RF3_48_PD344   DDR3 MSD_D3R_PDIFF_PDQSR cell  Z0=48-Ohm
MSD_D3RF3_34_PD393   DDR3 MSD_D3R_PDIFF_PDQSR cell  Z0=34-Ohm
MSD_D3RF3_40_PD393   DDR3 MSD_D3R_PDIFF_PDQSR cell  Z0=40-Ohm
MSD_D3RF3_48_PD393   DDR3 MSD_D3R_PDIFF_PDQSR cell  Z0=48-Ohm
MSD_D3RF3_34_PD458   DDR3 MSD_D3R_PDIFF_PDQSR cell  Z0=34-Ohm
MSD_D3RF3_40_PD458   DDR3 MSD_D3R_PDIFF_PDQSR cell  Z0=40-Ohm
MSD_D3RF3_48_PD458   DDR3 MSD_D3R_PDIFF_PDQSR cell  Z0=48-Ohm
MSD_D3RF3_34_PD500   DDR3 MSD_D3R_PDIFF_PDQSR cell  Z0=34-Ohm
MSD_D3RF3_40_PD500   DDR3 MSD_D3R_PDIFF_PDQSR cell  Z0=40-Ohm
MSD_D3RF3_48_PD500   DDR3 MSD_D3R_PDIFF_PDQSR cell  Z0=48-Ohm
MSD_D3RF3_34_PD550   DDR3 MSD_D3R_PDIFF_PDQSR cell  Z0=34-Ohm
MSD_D3RF3_40_PD550   DDR3 MSD_D3R_PDIFF_PDQSR cell  Z0=40-Ohm
MSD_D3RF3_48_PD550   DDR3 MSD_D3R_PDIFF_PDQSR cell  Z0=48-Ohm
MSD_D3RF3_34_PD611   DDR3 MSD_D3R_PDIFF_PDQSR cell  Z0=34-Ohm
MSD_D3RF3_40_PD611   DDR3 MSD_D3R_PDIFF_PDQSR cell  Z0=40-Ohm
MSD_D3RF3_48_PD611   DDR3 MSD_D3R_PDIFF_PDQSR cell  Z0=48-Ohm
MSD_D3RF3_34_PD688   DDR3 MSD_D3R_PDIFF_PDQSR cell  Z0=34-Ohm
MSD_D3RF3_40_PD688   DDR3 MSD_D3R_PDIFF_PDQSR cell  Z0=40-Ohm
MSD_D3RF3_48_PD688   DDR3 MSD_D3R_PDIFF_PDQSR cell  Z0=48-Ohm
MSD_D3RF3_34_PU344   DDR3 MSD_D3R_PDIFF_PDQSR cell  Z0=34-Ohm
MSD_D3RF3_40_PU344   DDR3 MSD_D3R_PDIFF_PDQSR cell  Z0=40-Ohm
MSD_D3RF3_48_PU344   DDR3 MSD_D3R_PDIFF_PDQSR cell  Z0=48-Ohm
MSD_D3RF3_34_PU393   DDR3 MSD_D3R_PDIFF_PDQSR cell  Z0=34-Ohm
MSD_D3RF3_40_PU393   DDR3 MSD_D3R_PDIFF_PDQSR cell  Z0=40-Ohm
MSD_D3RF3_48_PU393   DDR3 MSD_D3R_PDIFF_PDQSR cell  Z0=48-Ohm
MSD_D3RF3_34_PU458   DDR3 MSD_D3R_PDIFF_PDQSR cell  Z0=34-Ohm
MSD_D3RF3_40_PU458   DDR3 MSD_D3R_PDIFF_PDQSR cell  Z0=40-Ohm
MSD_D3RF3_48_PU458   DDR3 MSD_D3R_PDIFF_PDQSR cell  Z0=48-Ohm
MSD_D3RF3_34_PU500   DDR3 MSD_D3R_PDIFF_PDQSR cell  Z0=34-Ohm
MSD_D3RF3_40_PU500   DDR3 MSD_D3R_PDIFF_PDQSR cell  Z0=40-Ohm
MSD_D3RF3_48_PU500   DDR3 MSD_D3R_PDIFF_PDQSR cell  Z0=48-Ohm
MSD_D3RF3_34_PU550   DDR3 MSD_D3R_PDIFF_PDQSR cell  Z0=34-Ohm
MSD_D3RF3_40_PU550   DDR3 MSD_D3R_PDIFF_PDQSR cell  Z0=40-Ohm
MSD_D3RF3_48_PU550   DDR3 MSD_D3R_PDIFF_PDQSR cell  Z0=48-Ohm
MSD_D3RF3_34_PU611   DDR3 MSD_D3R_PDIFF_PDQSR cell  Z0=34-Ohm
MSD_D3RF3_40_PU611   DDR3 MSD_D3R_PDIFF_PDQSR cell  Z0=40-Ohm
MSD_D3RF3_48_PU611   DDR3 MSD_D3R_PDIFF_PDQSR cell  Z0=48-Ohm
MSD_D3RF3_34_PU688   DDR3 MSD_D3R_PDIFF_PDQSR cell  Z0=34-Ohm
MSD_D3RF3_40_PU688   DDR3 MSD_D3R_PDIFF_PDQSR cell  Z0=40-Ohm
MSD_D3RF3_48_PU688   DDR3 MSD_D3R_PDIFF_PDQSR cell  Z0=48-Ohm
MSD_D3RF3_34_PWRDWN   DDR3 MSD_D3R_PDIFF_PDQSR cell  Z0=34-Ohm
MSD_D3RF3_40_PWRDWN   DDR3 MSD_D3R_PDIFF_PDQSR cell  Z0=40-Ohm
MSD_D3RF3_48_PWRDWN   DDR3 MSD_D3R_PDIFF_PDQSR cell  Z0=48-Ohm
MSD_D3RF3L_34_OPEN   DDR3L MSD_D3R_PDIFF_PDQSR cell  Z0=34-Ohm
MSD_D3RF3L_40_OPEN   DDR3L MSD_D3R_PDIFF_PDQSR cell  Z0=40-Ohm
MSD_D3RF3L_48_OPEN   DDR3L MSD_D3R_PDIFF_PDQSR cell  Z0=48-Ohm
MSD_D3RF3L_34_PD344   DDR3L MSD_D3R_PDIFF_PDQSR cell  Z0=34-Ohm
MSD_D3RF3L_40_PD344   DDR3L MSD_D3R_PDIFF_PDQSR cell  Z0=40-Ohm
MSD_D3RF3L_48_PD344   DDR3L MSD_D3R_PDIFF_PDQSR cell  Z0=48-Ohm
MSD_D3RF3L_34_PD393   DDR3L MSD_D3R_PDIFF_PDQSR cell  Z0=34-Ohm
MSD_D3RF3L_40_PD393   DDR3L MSD_D3R_PDIFF_PDQSR cell  Z0=40-Ohm
MSD_D3RF3L_48_PD393   DDR3L MSD_D3R_PDIFF_PDQSR cell  Z0=48-Ohm
MSD_D3RF3L_34_PD458   DDR3L MSD_D3R_PDIFF_PDQSR cell  Z0=34-Ohm
MSD_D3RF3L_40_PD458   DDR3L MSD_D3R_PDIFF_PDQSR cell  Z0=40-Ohm
MSD_D3RF3L_48_PD458   DDR3L MSD_D3R_PDIFF_PDQSR cell  Z0=48-Ohm
MSD_D3RF3L_34_PD500   DDR3L MSD_D3R_PDIFF_PDQSR cell  Z0=34-Ohm
MSD_D3RF3L_40_PD500   DDR3L MSD_D3R_PDIFF_PDQSR cell  Z0=40-Ohm
MSD_D3RF3L_48_PD500   DDR3L MSD_D3R_PDIFF_PDQSR cell  Z0=48-Ohm
MSD_D3RF3L_34_PD550   DDR3L MSD_D3R_PDIFF_PDQSR cell  Z0=34-Ohm
MSD_D3RF3L_40_PD550   DDR3L MSD_D3R_PDIFF_PDQSR cell  Z0=40-Ohm
MSD_D3RF3L_48_PD550   DDR3L MSD_D3R_PDIFF_PDQSR cell  Z0=48-Ohm
MSD_D3RF3L_34_PD611   DDR3L MSD_D3R_PDIFF_PDQSR cell  Z0=34-Ohm
MSD_D3RF3L_40_PD611   DDR3L MSD_D3R_PDIFF_PDQSR cell  Z0=40-Ohm
MSD_D3RF3L_48_PD611   DDR3L MSD_D3R_PDIFF_PDQSR cell  Z0=48-Ohm
MSD_D3RF3L_34_PD688   DDR3L MSD_D3R_PDIFF_PDQSR cell  Z0=34-Ohm
MSD_D3RF3L_40_PD688   DDR3L MSD_D3R_PDIFF_PDQSR cell  Z0=40-Ohm
MSD_D3RF3L_48_PD688   DDR3L MSD_D3R_PDIFF_PDQSR cell  Z0=48-Ohm
MSD_D3RF3L_34_PU344   DDR3L MSD_D3R_PDIFF_PDQSR cell  Z0=34-Ohm
MSD_D3RF3L_40_PU344   DDR3L MSD_D3R_PDIFF_PDQSR cell  Z0=40-Ohm
MSD_D3RF3L_48_PU344   DDR3L MSD_D3R_PDIFF_PDQSR cell  Z0=48-Ohm
MSD_D3RF3L_34_PU393   DDR3L MSD_D3R_PDIFF_PDQSR cell  Z0=34-Ohm
MSD_D3RF3L_40_PU393   DDR3L MSD_D3R_PDIFF_PDQSR cell  Z0=40-Ohm
MSD_D3RF3L_48_PU393   DDR3L MSD_D3R_PDIFF_PDQSR cell  Z0=48-Ohm
MSD_D3RF3L_34_PU458   DDR3L MSD_D3R_PDIFF_PDQSR cell  Z0=34-Ohm
MSD_D3RF3L_40_PU458   DDR3L MSD_D3R_PDIFF_PDQSR cell  Z0=40-Ohm
MSD_D3RF3L_48_PU458   DDR3L MSD_D3R_PDIFF_PDQSR cell  Z0=48-Ohm
MSD_D3RF3L_34_PU500   DDR3L MSD_D3R_PDIFF_PDQSR cell  Z0=34-Ohm
MSD_D3RF3L_40_PU500   DDR3L MSD_D3R_PDIFF_PDQSR cell  Z0=40-Ohm
MSD_D3RF3L_48_PU500   DDR3L MSD_D3R_PDIFF_PDQSR cell  Z0=48-Ohm
MSD_D3RF3L_34_PU550   DDR3L MSD_D3R_PDIFF_PDQSR cell  Z0=34-Ohm
MSD_D3RF3L_40_PU550   DDR3L MSD_D3R_PDIFF_PDQSR cell  Z0=40-Ohm
MSD_D3RF3L_48_PU550   DDR3L MSD_D3R_PDIFF_PDQSR cell  Z0=48-Ohm
MSD_D3RF3L_34_PU611   DDR3L MSD_D3R_PDIFF_PDQSR cell  Z0=34-Ohm
MSD_D3RF3L_40_PU611   DDR3L MSD_D3R_PDIFF_PDQSR cell  Z0=40-Ohm
MSD_D3RF3L_48_PU611   DDR3L MSD_D3R_PDIFF_PDQSR cell  Z0=48-Ohm
MSD_D3RF3L_34_PU688   DDR3L MSD_D3R_PDIFF_PDQSR cell  Z0=34-Ohm
MSD_D3RF3L_40_PU688   DDR3L MSD_D3R_PDIFF_PDQSR cell  Z0=40-Ohm
MSD_D3RF3L_48_PU688   DDR3L MSD_D3R_PDIFF_PDQSR cell  Z0=48-Ohm
MSD_D3RF3L_34_PWRDWN   DDR3L MSD_D3R_PDIFF_PDQSR cell  Z0=34-Ohm
MSD_D3RF3L_40_PWRDWN   DDR3L MSD_D3R_PDIFF_PDQSR cell  Z0=40-Ohm
MSD_D3RF3L_48_PWRDWN   DDR3L MSD_D3R_PDIFF_PDQSR cell  Z0=48-Ohm
MSD_D3RFL2_34_OPEN   LPDDR2 MSD_D3R_PDIFF_PDQSR cell  Z0=34-Ohm
MSD_D3RFL2_40_OPEN   LPDDR2 MSD_D3R_PDIFF_PDQSR cell  Z0=40-Ohm
MSD_D3RFL2_48_OPEN   LPDDR2 MSD_D3R_PDIFF_PDQSR cell  Z0=48-Ohm
MSD_D3RFL2_60_OPEN   LPDDR2 MSD_D3R_PDIFF_PDQSR cell  Z0=60-Ohm
MSD_D3RFL2_80_OPEN   LPDDR2 MSD_D3R_PDIFF_PDQSR cell  Z0=80-Ohm
MSD_D3RFL_48_OPEN   LPDDR MSD_D3R_PDIFF_PDQSR cell  Z0=48-Ohm
MSD_D3RFL2_34_PD344   LPDDR2 MSD_D3R_PDIFF_PDQSR cell  Z0=34-Ohm
MSD_D3RFL2_40_PD344   LPDDR2 MSD_D3R_PDIFF_PDQSR cell  Z0=40-Ohm
MSD_D3RFL2_48_PD344   LPDDR2 MSD_D3R_PDIFF_PDQSR cell  Z0=48-Ohm
MSD_D3RFL2_60_PD344   LPDDR2 MSD_D3R_PDIFF_PDQSR cell  Z0=60-Ohm
MSD_D3RFL2_80_PD344   LPDDR2 MSD_D3R_PDIFF_PDQSR cell  Z0=80-Ohm
MSD_D3RFL_48_PD344   LPDDR MSD_D3R_PDIFF_PDQSR cell  Z0=48-Ohm
MSD_D3RFL2_34_PD393   LPDDR2 MSD_D3R_PDIFF_PDQSR cell  Z0=34-Ohm
MSD_D3RFL2_40_PD393   LPDDR2 MSD_D3R_PDIFF_PDQSR cell  Z0=40-Ohm
MSD_D3RFL2_48_PD393   LPDDR2 MSD_D3R_PDIFF_PDQSR cell  Z0=48-Ohm
MSD_D3RFL2_60_PD393   LPDDR2 MSD_D3R_PDIFF_PDQSR cell  Z0=60-Ohm
MSD_D3RFL2_80_PD393   LPDDR2 MSD_D3R_PDIFF_PDQSR cell  Z0=80-Ohm
MSD_D3RFL_48_PD393   LPDDR MSD_D3R_PDIFF_PDQSR cell  Z0=48-Ohm
MSD_D3RFL2_34_PD458   LPDDR2 MSD_D3R_PDIFF_PDQSR cell  Z0=34-Ohm
MSD_D3RFL2_40_PD458   LPDDR2 MSD_D3R_PDIFF_PDQSR cell  Z0=40-Ohm
MSD_D3RFL2_48_PD458   LPDDR2 MSD_D3R_PDIFF_PDQSR cell  Z0=48-Ohm
MSD_D3RFL2_60_PD458   LPDDR2 MSD_D3R_PDIFF_PDQSR cell  Z0=60-Ohm
MSD_D3RFL2_80_PD458   LPDDR2 MSD_D3R_PDIFF_PDQSR cell  Z0=80-Ohm
MSD_D3RFL_48_PD458   LPDDR MSD_D3R_PDIFF_PDQSR cell  Z0=48-Ohm
MSD_D3RFL2_34_PD500   LPDDR2 MSD_D3R_PDIFF_PDQSR cell  Z0=34-Ohm
MSD_D3RFL2_40_PD500   LPDDR2 MSD_D3R_PDIFF_PDQSR cell  Z0=40-Ohm
MSD_D3RFL2_48_PD500   LPDDR2 MSD_D3R_PDIFF_PDQSR cell  Z0=48-Ohm
MSD_D3RFL2_60_PD500   LPDDR2 MSD_D3R_PDIFF_PDQSR cell  Z0=60-Ohm
MSD_D3RFL2_80_PD500   LPDDR2 MSD_D3R_PDIFF_PDQSR cell  Z0=80-Ohm
MSD_D3RFL_48_PD500   LPDDR MSD_D3R_PDIFF_PDQSR cell  Z0=48-Ohm
MSD_D3RFL2_34_PD550   LPDDR2 MSD_D3R_PDIFF_PDQSR cell  Z0=34-Ohm
MSD_D3RFL2_40_PD550   LPDDR2 MSD_D3R_PDIFF_PDQSR cell  Z0=40-Ohm
MSD_D3RFL2_48_PD550   LPDDR2 MSD_D3R_PDIFF_PDQSR cell  Z0=48-Ohm
MSD_D3RFL2_60_PD550   LPDDR2 MSD_D3R_PDIFF_PDQSR cell  Z0=60-Ohm
MSD_D3RFL2_80_PD550   LPDDR2 MSD_D3R_PDIFF_PDQSR cell  Z0=80-Ohm
MSD_D3RFL_48_PD550   LPDDR MSD_D3R_PDIFF_PDQSR cell  Z0=48-Ohm
MSD_D3RFL2_34_PD611   LPDDR2 MSD_D3R_PDIFF_PDQSR cell  Z0=34-Ohm
MSD_D3RFL2_40_PD611   LPDDR2 MSD_D3R_PDIFF_PDQSR cell  Z0=40-Ohm
MSD_D3RFL2_48_PD611   LPDDR2 MSD_D3R_PDIFF_PDQSR cell  Z0=48-Ohm
MSD_D3RFL2_60_PD611   LPDDR2 MSD_D3R_PDIFF_PDQSR cell  Z0=60-Ohm
MSD_D3RFL2_80_PD611   LPDDR2 MSD_D3R_PDIFF_PDQSR cell  Z0=80-Ohm
MSD_D3RFL_48_PD611   LPDDR MSD_D3R_PDIFF_PDQSR cell  Z0=48-Ohm
MSD_D3RFL2_34_PD688   LPDDR2 MSD_D3R_PDIFF_PDQSR cell  Z0=34-Ohm
MSD_D3RFL2_40_PD688   LPDDR2 MSD_D3R_PDIFF_PDQSR cell  Z0=40-Ohm
MSD_D3RFL2_48_PD688   LPDDR2 MSD_D3R_PDIFF_PDQSR cell  Z0=48-Ohm
MSD_D3RFL2_60_PD688   LPDDR2 MSD_D3R_PDIFF_PDQSR cell  Z0=60-Ohm
MSD_D3RFL2_80_PD688   LPDDR2 MSD_D3R_PDIFF_PDQSR cell  Z0=80-Ohm
MSD_D3RFL_48_PD688   LPDDR MSD_D3R_PDIFF_PDQSR cell  Z0=48-Ohm
MSD_D3RFL2_34_PU344   LPDDR2 MSD_D3R_PDIFF_PDQSR cell  Z0=34-Ohm
MSD_D3RFL2_40_PU344   LPDDR2 MSD_D3R_PDIFF_PDQSR cell  Z0=40-Ohm
MSD_D3RFL2_48_PU344   LPDDR2 MSD_D3R_PDIFF_PDQSR cell  Z0=48-Ohm
MSD_D3RFL2_60_PU344   LPDDR2 MSD_D3R_PDIFF_PDQSR cell  Z0=60-Ohm
MSD_D3RFL2_80_PU344   LPDDR2 MSD_D3R_PDIFF_PDQSR cell  Z0=80-Ohm
MSD_D3RFL_48_PU344   LPDDR MSD_D3R_PDIFF_PDQSR cell  Z0=48-Ohm
MSD_D3RFL2_34_PU393   LPDDR2 MSD_D3R_PDIFF_PDQSR cell  Z0=34-Ohm
MSD_D3RFL2_40_PU393   LPDDR2 MSD_D3R_PDIFF_PDQSR cell  Z0=40-Ohm
MSD_D3RFL2_48_PU393   LPDDR2 MSD_D3R_PDIFF_PDQSR cell  Z0=48-Ohm
MSD_D3RFL2_60_PU393   LPDDR2 MSD_D3R_PDIFF_PDQSR cell  Z0=60-Ohm
MSD_D3RFL2_80_PU393   LPDDR2 MSD_D3R_PDIFF_PDQSR cell  Z0=80-Ohm
MSD_D3RFL_48_PU393   LPDDR MSD_D3R_PDIFF_PDQSR cell  Z0=48-Ohm
MSD_D3RFL2_34_PU458   LPDDR2 MSD_D3R_PDIFF_PDQSR cell  Z0=34-Ohm
MSD_D3RFL2_40_PU458   LPDDR2 MSD_D3R_PDIFF_PDQSR cell  Z0=40-Ohm
MSD_D3RFL2_48_PU458   LPDDR2 MSD_D3R_PDIFF_PDQSR cell  Z0=48-Ohm
MSD_D3RFL2_60_PU458   LPDDR2 MSD_D3R_PDIFF_PDQSR cell  Z0=60-Ohm
MSD_D3RFL2_80_PU458   LPDDR2 MSD_D3R_PDIFF_PDQSR cell  Z0=80-Ohm
MSD_D3RFL_48_PU458   LPDDR MSD_D3R_PDIFF_PDQSR cell  Z0=48-Ohm
MSD_D3RFL2_34_PU500   LPDDR2 MSD_D3R_PDIFF_PDQSR cell  Z0=34-Ohm
MSD_D3RFL2_40_PU500   LPDDR2 MSD_D3R_PDIFF_PDQSR cell  Z0=40-Ohm
MSD_D3RFL2_48_PU500   LPDDR2 MSD_D3R_PDIFF_PDQSR cell  Z0=48-Ohm
MSD_D3RFL2_60_PU500   LPDDR2 MSD_D3R_PDIFF_PDQSR cell  Z0=60-Ohm
MSD_D3RFL2_80_PU500   LPDDR2 MSD_D3R_PDIFF_PDQSR cell  Z0=80-Ohm
MSD_D3RFL_48_PU500   LPDDR MSD_D3R_PDIFF_PDQSR cell  Z0=48-Ohm
MSD_D3RFL2_34_PU550   LPDDR2 MSD_D3R_PDIFF_PDQSR cell  Z0=34-Ohm
MSD_D3RFL2_40_PU550   LPDDR2 MSD_D3R_PDIFF_PDQSR cell  Z0=40-Ohm
MSD_D3RFL2_48_PU550   LPDDR2 MSD_D3R_PDIFF_PDQSR cell  Z0=48-Ohm
MSD_D3RFL2_60_PU550   LPDDR2 MSD_D3R_PDIFF_PDQSR cell  Z0=60-Ohm
MSD_D3RFL2_80_PU550   LPDDR2 MSD_D3R_PDIFF_PDQSR cell  Z0=80-Ohm
MSD_D3RFL_48_PU550   LPDDR MSD_D3R_PDIFF_PDQSR cell  Z0=48-Ohm
MSD_D3RFL2_34_PU611   LPDDR2 MSD_D3R_PDIFF_PDQSR cell  Z0=34-Ohm
MSD_D3RFL2_40_PU611   LPDDR2 MSD_D3R_PDIFF_PDQSR cell  Z0=40-Ohm
MSD_D3RFL2_48_PU611   LPDDR2 MSD_D3R_PDIFF_PDQSR cell  Z0=48-Ohm
MSD_D3RFL2_60_PU611   LPDDR2 MSD_D3R_PDIFF_PDQSR cell  Z0=60-Ohm
MSD_D3RFL2_80_PU611   LPDDR2 MSD_D3R_PDIFF_PDQSR cell  Z0=80-Ohm
MSD_D3RFL_48_PU611   LPDDR MSD_D3R_PDIFF_PDQSR cell  Z0=48-Ohm
MSD_D3RFL2_34_PU688   LPDDR2 MSD_D3R_PDIFF_PDQSR cell  Z0=34-Ohm
MSD_D3RFL2_40_PU688   LPDDR2 MSD_D3R_PDIFF_PDQSR cell  Z0=40-Ohm
MSD_D3RFL2_48_PU688   LPDDR2 MSD_D3R_PDIFF_PDQSR cell  Z0=48-Ohm
MSD_D3RFL2_60_PU688   LPDDR2 MSD_D3R_PDIFF_PDQSR cell  Z0=60-Ohm
MSD_D3RFL2_80_PU688   LPDDR2 MSD_D3R_PDIFF_PDQSR cell  Z0=80-Ohm
MSD_D3RFL_48_PU688   LPDDR MSD_D3R_PDIFF_PDQSR cell  Z0=48-Ohm
MSD_D3RFL2_34_PWRDWN   LPDDR2 MSD_D3R_PDIFF_PDQSR cell  Z0=34-Ohm
MSD_D3RFL2_40_PWRDWN   LPDDR2 MSD_D3R_PDIFF_PDQSR cell  Z0=40-Ohm
MSD_D3RFL2_48_PWRDWN   LPDDR2 MSD_D3R_PDIFF_PDQSR cell  Z0=48-Ohm
MSD_D3RFL2_60_PWRDWN   LPDDR2 MSD_D3R_PDIFF_PDQSR cell  Z0=60-Ohm
MSD_D3RFL2_80_PWRDWN   LPDDR2 MSD_D3R_PDIFF_PDQSR cell  Z0=80-Ohm
MSD_D3RFL_48_PWRDWN   LPDDR MSD_D3R_PDIFF_PDQSR cell  Z0=48-Ohm
MSD_D3RF2_ODT150_OPEN   DDR2 MSD_D3R_PDIFF_PDQSR cell 150-Ohm ODT Receiver
MSD_D3RF2_ODT50_OPEN   DDR2 MSD_D3R_PDIFF_PDQSR cell 50-Ohm ODT Receiver
MSD_D3RF2_ODT75_OPEN   DDR2 MSD_D3R_PDIFF_PDQSR cell 75-Ohm ODT Receiver
MSD_D3RF2_ODTOFF_OPEN   DDR2 MSD_D3R_PDIFF_PDQSR cell ODT off Receiver
MSD_D3RF2_ODT150_PD344   DDR2 MSD_D3R_PDIFF_PDQSR cell 150-Ohm ODT Receiver
MSD_D3RF2_ODT50_PD344   DDR2 MSD_D3R_PDIFF_PDQSR cell 50-Ohm ODT Receiver
MSD_D3RF2_ODT75_PD344   DDR2 MSD_D3R_PDIFF_PDQSR cell 75-Ohm ODT Receiver
MSD_D3RF2_ODTOFF_PD344   DDR2 MSD_D3R_PDIFF_PDQSR cell ODT off Receiver
MSD_D3RF2_ODT150_PD393   DDR2 MSD_D3R_PDIFF_PDQSR cell 150-Ohm ODT Receiver
MSD_D3RF2_ODT50_PD393   DDR2 MSD_D3R_PDIFF_PDQSR cell 50-Ohm ODT Receiver
MSD_D3RF2_ODT75_PD393   DDR2 MSD_D3R_PDIFF_PDQSR cell 75-Ohm ODT Receiver
MSD_D3RF2_ODTOFF_PD393   DDR2 MSD_D3R_PDIFF_PDQSR cell ODT off Receiver
MSD_D3RF2_ODT150_PD458   DDR2 MSD_D3R_PDIFF_PDQSR cell 150-Ohm ODT Receiver
MSD_D3RF2_ODT50_PD458   DDR2 MSD_D3R_PDIFF_PDQSR cell 50-Ohm ODT Receiver
MSD_D3RF2_ODT75_PD458   DDR2 MSD_D3R_PDIFF_PDQSR cell 75-Ohm ODT Receiver
MSD_D3RF2_ODTOFF_PD458   DDR2 MSD_D3R_PDIFF_PDQSR cell ODT off Receiver
MSD_D3RF2_ODT150_PD500   DDR2 MSD_D3R_PDIFF_PDQSR cell 150-Ohm ODT Receiver
MSD_D3RF2_ODT50_PD500   DDR2 MSD_D3R_PDIFF_PDQSR cell 50-Ohm ODT Receiver
MSD_D3RF2_ODT75_PD500   DDR2 MSD_D3R_PDIFF_PDQSR cell 75-Ohm ODT Receiver
MSD_D3RF2_ODTOFF_PD500   DDR2 MSD_D3R_PDIFF_PDQSR cell ODT off Receiver
MSD_D3RF2_ODT150_PD550   DDR2 MSD_D3R_PDIFF_PDQSR cell 150-Ohm ODT Receiver
MSD_D3RF2_ODT50_PD550   DDR2 MSD_D3R_PDIFF_PDQSR cell 50-Ohm ODT Receiver
MSD_D3RF2_ODT75_PD550   DDR2 MSD_D3R_PDIFF_PDQSR cell 75-Ohm ODT Receiver
MSD_D3RF2_ODTOFF_PD550   DDR2 MSD_D3R_PDIFF_PDQSR cell ODT off Receiver
MSD_D3RF2_ODT150_PD611   DDR2 MSD_D3R_PDIFF_PDQSR cell 150-Ohm ODT Receiver
MSD_D3RF2_ODT50_PD611   DDR2 MSD_D3R_PDIFF_PDQSR cell 50-Ohm ODT Receiver
MSD_D3RF2_ODT75_PD611   DDR2 MSD_D3R_PDIFF_PDQSR cell 75-Ohm ODT Receiver
MSD_D3RF2_ODTOFF_PD611   DDR2 MSD_D3R_PDIFF_PDQSR cell ODT off Receiver
MSD_D3RF2_ODT150_PD688   DDR2 MSD_D3R_PDIFF_PDQSR cell 150-Ohm ODT Receiver
MSD_D3RF2_ODT50_PD688   DDR2 MSD_D3R_PDIFF_PDQSR cell 50-Ohm ODT Receiver
MSD_D3RF2_ODT75_PD688   DDR2 MSD_D3R_PDIFF_PDQSR cell 75-Ohm ODT Receiver
MSD_D3RF2_ODTOFF_PD688   DDR2 MSD_D3R_PDIFF_PDQSR cell ODT off Receiver
MSD_D3RF2_ODT150_PU344   DDR2 MSD_D3R_PDIFF_PDQSR cell 150-Ohm ODT Receiver
MSD_D3RF2_ODT50_PU344   DDR2 MSD_D3R_PDIFF_PDQSR cell 50-Ohm ODT Receiver
MSD_D3RF2_ODT75_PU344   DDR2 MSD_D3R_PDIFF_PDQSR cell 75-Ohm ODT Receiver
MSD_D3RF2_ODTOFF_PU344   DDR2 MSD_D3R_PDIFF_PDQSR cell ODT off Receiver
MSD_D3RF2_ODT150_PU393   DDR2 MSD_D3R_PDIFF_PDQSR cell 150-Ohm ODT Receiver
MSD_D3RF2_ODT50_PU393   DDR2 MSD_D3R_PDIFF_PDQSR cell 50-Ohm ODT Receiver
MSD_D3RF2_ODT75_PU393   DDR2 MSD_D3R_PDIFF_PDQSR cell 75-Ohm ODT Receiver
MSD_D3RF2_ODTOFF_PU393   DDR2 MSD_D3R_PDIFF_PDQSR cell ODT off Receiver
MSD_D3RF2_ODT150_PU458   DDR2 MSD_D3R_PDIFF_PDQSR cell 150-Ohm ODT Receiver
MSD_D3RF2_ODT50_PU458   DDR2 MSD_D3R_PDIFF_PDQSR cell 50-Ohm ODT Receiver
MSD_D3RF2_ODT75_PU458   DDR2 MSD_D3R_PDIFF_PDQSR cell 75-Ohm ODT Receiver
MSD_D3RF2_ODTOFF_PU458   DDR2 MSD_D3R_PDIFF_PDQSR cell ODT off Receiver
MSD_D3RF2_ODT150_PU500   DDR2 MSD_D3R_PDIFF_PDQSR cell 150-Ohm ODT Receiver
MSD_D3RF2_ODT50_PU500   DDR2 MSD_D3R_PDIFF_PDQSR cell 50-Ohm ODT Receiver
MSD_D3RF2_ODT75_PU500   DDR2 MSD_D3R_PDIFF_PDQSR cell 75-Ohm ODT Receiver
MSD_D3RF2_ODTOFF_PU500   DDR2 MSD_D3R_PDIFF_PDQSR cell ODT off Receiver
MSD_D3RF2_ODT150_PU550   DDR2 MSD_D3R_PDIFF_PDQSR cell 150-Ohm ODT Receiver
MSD_D3RF2_ODT50_PU550   DDR2 MSD_D3R_PDIFF_PDQSR cell 50-Ohm ODT Receiver
MSD_D3RF2_ODT75_PU550   DDR2 MSD_D3R_PDIFF_PDQSR cell 75-Ohm ODT Receiver
MSD_D3RF2_ODTOFF_PU550   DDR2 MSD_D3R_PDIFF_PDQSR cell ODT off Receiver
MSD_D3RF2_ODT150_PU611   DDR2 MSD_D3R_PDIFF_PDQSR cell 150-Ohm ODT Receiver
MSD_D3RF2_ODT50_PU611   DDR2 MSD_D3R_PDIFF_PDQSR cell 50-Ohm ODT Receiver
MSD_D3RF2_ODT75_PU611   DDR2 MSD_D3R_PDIFF_PDQSR cell 75-Ohm ODT Receiver
MSD_D3RF2_ODTOFF_PU611   DDR2 MSD_D3R_PDIFF_PDQSR cell ODT off Receiver
MSD_D3RF2_ODT150_PU688   DDR2 MSD_D3R_PDIFF_PDQSR cell 150-Ohm ODT Receiver
MSD_D3RF2_ODT50_PU688   DDR2 MSD_D3R_PDIFF_PDQSR cell 50-Ohm ODT Receiver
MSD_D3RF2_ODT75_PU688   DDR2 MSD_D3R_PDIFF_PDQSR cell 75-Ohm ODT Receiver
MSD_D3RF2_ODTOFF_PU688   DDR2 MSD_D3R_PDIFF_PDQSR cell ODT off Receiver
MSD_D3RF2_ODT150_PWRDWN   DDR2 MSD_D3R_PDIFF_PDQSR cell 150-Ohm ODT Receiver
MSD_D3RF2_ODT50_PWRDWN   DDR2 MSD_D3R_PDIFF_PDQSR cell 50-Ohm ODT Receiver
MSD_D3RF2_ODT75_PWRDWN   DDR2 MSD_D3R_PDIFF_PDQSR cell 75-Ohm ODT Receiver
MSD_D3RF2_ODTOFF_PWRDWN   DDR2 MSD_D3R_PDIFF_PDQSR cell ODT off Receiver
MSD_D3RF3_ODT120_OPEN   DDR3 MSD_D3R_PDIFF_PDQSR cell 120-Ohm ODT Receiver
MSD_D3RF3_ODT40_OPEN   DDR3 MSD_D3R_PDIFF_PDQSR cell 40-Ohm ODT Receiver
MSD_D3RF3_ODT60_OPEN   DDR3 MSD_D3R_PDIFF_PDQSR cell 60-Ohm ODT Receiver
MSD_D3RF3_ODTOFF_OPEN   DDR3 MSD_D3R_PDIFF_PDQSR cell ODT off Receiver
MSD_D3RF3_ODT120_PD344   DDR3 MSD_D3R_PDIFF_PDQSR cell 120-Ohm ODT Receiver
MSD_D3RF3_ODT40_PD344   DDR3 MSD_D3R_PDIFF_PDQSR cell 40-Ohm ODT Receiver
MSD_D3RF3_ODT60_PD344   DDR3 MSD_D3R_PDIFF_PDQSR cell 60-Ohm ODT Receiver
MSD_D3RF3_ODTOFF_PD344   DDR3 MSD_D3R_PDIFF_PDQSR cell ODT off Receiver
MSD_D3RF3_ODT120_PD393   DDR3 MSD_D3R_PDIFF_PDQSR cell 120-Ohm ODT Receiver
MSD_D3RF3_ODT40_PD393   DDR3 MSD_D3R_PDIFF_PDQSR cell 40-Ohm ODT Receiver
MSD_D3RF3_ODT60_PD393   DDR3 MSD_D3R_PDIFF_PDQSR cell 60-Ohm ODT Receiver
MSD_D3RF3_ODTOFF_PD393   DDR3 MSD_D3R_PDIFF_PDQSR cell ODT off Receiver
MSD_D3RF3_ODT120_PD458   DDR3 MSD_D3R_PDIFF_PDQSR cell 120-Ohm ODT Receiver
MSD_D3RF3_ODT40_PD458   DDR3 MSD_D3R_PDIFF_PDQSR cell 40-Ohm ODT Receiver
MSD_D3RF3_ODT60_PD458   DDR3 MSD_D3R_PDIFF_PDQSR cell 60-Ohm ODT Receiver
MSD_D3RF3_ODTOFF_PD458   DDR3 MSD_D3R_PDIFF_PDQSR cell ODT off Receiver
MSD_D3RF3_ODT120_PD500   DDR3 MSD_D3R_PDIFF_PDQSR cell 120-Ohm ODT Receiver
MSD_D3RF3_ODT40_PD500   DDR3 MSD_D3R_PDIFF_PDQSR cell 40-Ohm ODT Receiver
MSD_D3RF3_ODT60_PD500   DDR3 MSD_D3R_PDIFF_PDQSR cell 60-Ohm ODT Receiver
MSD_D3RF3_ODTOFF_PD500   DDR3 MSD_D3R_PDIFF_PDQSR cell ODT off Receiver
MSD_D3RF3_ODT120_PD550   DDR3 MSD_D3R_PDIFF_PDQSR cell 120-Ohm ODT Receiver
MSD_D3RF3_ODT40_PD550   DDR3 MSD_D3R_PDIFF_PDQSR cell 40-Ohm ODT Receiver
MSD_D3RF3_ODT60_PD550   DDR3 MSD_D3R_PDIFF_PDQSR cell 60-Ohm ODT Receiver
MSD_D3RF3_ODTOFF_PD550   DDR3 MSD_D3R_PDIFF_PDQSR cell ODT off Receiver
MSD_D3RF3_ODT120_PD611   DDR3 MSD_D3R_PDIFF_PDQSR cell 120-Ohm ODT Receiver
MSD_D3RF3_ODT40_PD611   DDR3 MSD_D3R_PDIFF_PDQSR cell 40-Ohm ODT Receiver
MSD_D3RF3_ODT60_PD611   DDR3 MSD_D3R_PDIFF_PDQSR cell 60-Ohm ODT Receiver
MSD_D3RF3_ODTOFF_PD611   DDR3 MSD_D3R_PDIFF_PDQSR cell ODT off Receiver
MSD_D3RF3_ODT120_PD688   DDR3 MSD_D3R_PDIFF_PDQSR cell 120-Ohm ODT Receiver
MSD_D3RF3_ODT40_PD688   DDR3 MSD_D3R_PDIFF_PDQSR cell 40-Ohm ODT Receiver
MSD_D3RF3_ODT60_PD688   DDR3 MSD_D3R_PDIFF_PDQSR cell 60-Ohm ODT Receiver
MSD_D3RF3_ODTOFF_PD688   DDR3 MSD_D3R_PDIFF_PDQSR cell ODT off Receiver
MSD_D3RF3_ODT120_PU344   DDR3 MSD_D3R_PDIFF_PDQSR cell 120-Ohm ODT Receiver
MSD_D3RF3_ODT40_PU344   DDR3 MSD_D3R_PDIFF_PDQSR cell 40-Ohm ODT Receiver
MSD_D3RF3_ODT60_PU344   DDR3 MSD_D3R_PDIFF_PDQSR cell 60-Ohm ODT Receiver
MSD_D3RF3_ODTOFF_PU344   DDR3 MSD_D3R_PDIFF_PDQSR cell ODT off Receiver
MSD_D3RF3_ODT120_PU393   DDR3 MSD_D3R_PDIFF_PDQSR cell 120-Ohm ODT Receiver
MSD_D3RF3_ODT40_PU393   DDR3 MSD_D3R_PDIFF_PDQSR cell 40-Ohm ODT Receiver
MSD_D3RF3_ODT60_PU393   DDR3 MSD_D3R_PDIFF_PDQSR cell 60-Ohm ODT Receiver
MSD_D3RF3_ODTOFF_PU393   DDR3 MSD_D3R_PDIFF_PDQSR cell ODT off Receiver
MSD_D3RF3_ODT120_PU458   DDR3 MSD_D3R_PDIFF_PDQSR cell 120-Ohm ODT Receiver
MSD_D3RF3_ODT40_PU458   DDR3 MSD_D3R_PDIFF_PDQSR cell 40-Ohm ODT Receiver
MSD_D3RF3_ODT60_PU458   DDR3 MSD_D3R_PDIFF_PDQSR cell 60-Ohm ODT Receiver
MSD_D3RF3_ODTOFF_PU458   DDR3 MSD_D3R_PDIFF_PDQSR cell ODT off Receiver
MSD_D3RF3_ODT120_PU500   DDR3 MSD_D3R_PDIFF_PDQSR cell 120-Ohm ODT Receiver
MSD_D3RF3_ODT40_PU500   DDR3 MSD_D3R_PDIFF_PDQSR cell 40-Ohm ODT Receiver
MSD_D3RF3_ODT60_PU500   DDR3 MSD_D3R_PDIFF_PDQSR cell 60-Ohm ODT Receiver
MSD_D3RF3_ODTOFF_PU500   DDR3 MSD_D3R_PDIFF_PDQSR cell ODT off Receiver
MSD_D3RF3_ODT120_PU550   DDR3 MSD_D3R_PDIFF_PDQSR cell 120-Ohm ODT Receiver
MSD_D3RF3_ODT40_PU550   DDR3 MSD_D3R_PDIFF_PDQSR cell 40-Ohm ODT Receiver
MSD_D3RF3_ODT60_PU550   DDR3 MSD_D3R_PDIFF_PDQSR cell 60-Ohm ODT Receiver
MSD_D3RF3_ODTOFF_PU550   DDR3 MSD_D3R_PDIFF_PDQSR cell ODT off Receiver
MSD_D3RF3_ODT120_PU611   DDR3 MSD_D3R_PDIFF_PDQSR cell 120-Ohm ODT Receiver
MSD_D3RF3_ODT40_PU611   DDR3 MSD_D3R_PDIFF_PDQSR cell 40-Ohm ODT Receiver
MSD_D3RF3_ODT60_PU611   DDR3 MSD_D3R_PDIFF_PDQSR cell 60-Ohm ODT Receiver
MSD_D3RF3_ODTOFF_PU611   DDR3 MSD_D3R_PDIFF_PDQSR cell ODT off Receiver
MSD_D3RF3_ODT120_PU688   DDR3 MSD_D3R_PDIFF_PDQSR cell 120-Ohm ODT Receiver
MSD_D3RF3_ODT40_PU688   DDR3 MSD_D3R_PDIFF_PDQSR cell 40-Ohm ODT Receiver
MSD_D3RF3_ODT60_PU688   DDR3 MSD_D3R_PDIFF_PDQSR cell 60-Ohm ODT Receiver
MSD_D3RF3_ODTOFF_PU688   DDR3 MSD_D3R_PDIFF_PDQSR cell ODT off Receiver
MSD_D3RF3_ODT120_PWRDWN   DDR3 MSD_D3R_PDIFF_PDQSR cell 120-Ohm ODT Receiver
MSD_D3RF3_ODT40_PWRDWN   DDR3 MSD_D3R_PDIFF_PDQSR cell 40-Ohm ODT Receiver
MSD_D3RF3_ODT60_PWRDWN   DDR3 MSD_D3R_PDIFF_PDQSR cell 60-Ohm ODT Receiver
MSD_D3RF3_ODTOFF_PWRDWN   DDR3 MSD_D3R_PDIFF_PDQSR cell ODT off Receiver
MSD_D3RF3L_ODT120_OPEN   DDR3L MSD_D3R_PDIFF_PDQSR cell 120-Ohm ODT Receiver
MSD_D3RF3L_ODT40_OPEN   DDR3L MSD_D3R_PDIFF_PDQSR cell 40-Ohm ODT Receiver
MSD_D3RF3L_ODT60_OPEN   DDR3L MSD_D3R_PDIFF_PDQSR cell 60-Ohm ODT Receiver
MSD_D3RF3L_ODTOFF_OPEN   DDR3L MSD_D3R_PDIFF_PDQSR cell ODT off Receiver
MSD_D3RF3L_ODT120_PD344   DDR3L MSD_D3R_PDIFF_PDQSR cell 120-Ohm ODT Receiver
MSD_D3RF3L_ODT40_PD344   DDR3L MSD_D3R_PDIFF_PDQSR cell 40-Ohm ODT Receiver
MSD_D3RF3L_ODT60_PD344   DDR3L MSD_D3R_PDIFF_PDQSR cell 60-Ohm ODT Receiver
MSD_D3RF3L_ODTOFF_PD344   DDR3L MSD_D3R_PDIFF_PDQSR cell ODT off Receiver
MSD_D3RF3L_ODT120_PD393   DDR3L MSD_D3R_PDIFF_PDQSR cell 120-Ohm ODT Receiver
MSD_D3RF3L_ODT40_PD393   DDR3L MSD_D3R_PDIFF_PDQSR cell 40-Ohm ODT Receiver
MSD_D3RF3L_ODT60_PD393   DDR3L MSD_D3R_PDIFF_PDQSR cell 60-Ohm ODT Receiver
MSD_D3RF3L_ODTOFF_PD393   DDR3L MSD_D3R_PDIFF_PDQSR cell ODT off Receiver
MSD_D3RF3L_ODT120_PD458   DDR3L MSD_D3R_PDIFF_PDQSR cell 120-Ohm ODT Receiver
MSD_D3RF3L_ODT40_PD458   DDR3L MSD_D3R_PDIFF_PDQSR cell 40-Ohm ODT Receiver
MSD_D3RF3L_ODT60_PD458   DDR3L MSD_D3R_PDIFF_PDQSR cell 60-Ohm ODT Receiver
MSD_D3RF3L_ODTOFF_PD458   DDR3L MSD_D3R_PDIFF_PDQSR cell ODT off Receiver
MSD_D3RF3L_ODT120_PD500   DDR3L MSD_D3R_PDIFF_PDQSR cell 120-Ohm ODT Receiver
MSD_D3RF3L_ODT40_PD500   DDR3L MSD_D3R_PDIFF_PDQSR cell 40-Ohm ODT Receiver
MSD_D3RF3L_ODT60_PD500   DDR3L MSD_D3R_PDIFF_PDQSR cell 60-Ohm ODT Receiver
MSD_D3RF3L_ODTOFF_PD500   DDR3L MSD_D3R_PDIFF_PDQSR cell ODT off Receiver
MSD_D3RF3L_ODT120_PD550   DDR3L MSD_D3R_PDIFF_PDQSR cell 120-Ohm ODT Receiver
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| Models and submodels in the file (581): io8_ft_et_fs_1v2 (I/O), io8_ft_et_hs_1v2 (I/O), io8_ft_et_hslv_fs_1v2 (I/O), io8_ft_et_hslv_hs_1v2 (I/O), io8_ft_et_hslv_ls_1v2 (I/O), io8_ft_et_hslv_ms_1v2 (I/O), io8_ft_et_ls_1v2 (I/O), io8_ft_et_ms_1v2 (I/O), io8_ft_fs_1v2 (I/O), io8_ft_hs_1v2 (I/O), io8_ft_hslv_fs_1v2 (I/O), io8_ft_hslv_hs_1v2 (I/O), io8_ft_hslv_ls_1v2 (I/O), io8_ft_hslv_ms_1v2 (I/O), io8_ft_i2c_1v2 (I/O_open_drain), io8_ft_i2c_hslv_1v2 (I/O_open_drain), io8_ft_ls_1v2 (I/O), io8_ft_ms_1v2 (I/O), isudqf_ft_1v2 (Input), io8_ft_et_fs_1v8 (I/O), io8_ft_et_hs_1v8 (I/O), io8_ft_et_hslv_fs_1v8 (I/O), io8_ft_et_hslv_hs_1v8 (I/O), io8_ft_et_hslv_ls_1v8 (I/O), io8_ft_et_hslv_ms_1v8 (I/O), io8_ft_et_ls_1v8 (I/O), io8_ft_et_ms_1v8 (I/O), io8_ft_fs_1v8 (I/O), io8_ft_hs_1v8 (I/O), io8_ft_hslv_fs_1v8 (I/O), io8_ft_hslv_hs_1v8 (I/O), io8_ft_hslv_ls_1v8 (I/O), io8_ft_hslv_ms_1v8 (I/O), io8_ft_i2c_1v8 (I/O_open_drain), io8_ft_i2c_hslv_1v8 (I/O_open_drain), io8_ft_ls_1v8 (I/O), io8_ft_ms_1v8 (I/O), isudqf_ft_1v8 (Input), io8_ft_et_hslv_fs_2v5 (I/O), io8_ft_et_hslv_hs_2v5 (I/O), io8_ft_et_hslv_ls_2v5 (I/O), io8_ft_et_hslv_ms_2v5 (I/O), io8_ft_hslv_fs_2v5 (I/O), io8_ft_hslv_hs_2v5 (I/O), io8_ft_hslv_ls_2v5 (I/O), io8_ft_hslv_ms_2v5 (I/O), io8_ft_i2c_hslv_2v5 (I/O_open_drain), io8_ft_et_fs_3v3 (I/O), io8_ft_et_hs_3v3 (I/O), io8_ft_et_ls_3v3 (I/O), io8_ft_et_ms_3v3 (I/O), io8_ft_fs_3v3 (I/O), io8_ft_hs_3v3 (I/O), io8_ft_i2c_3v3 (I/O_open_drain), io8_ft_ls_3v3 (I/O), io8_ft_ms_3v3 (I/O), io8usb_ft_hs_3v3 (I/O), io8usb_ft_ls_3v3 (I/O), isudqf_ft_3v3 (Input), MSD_D3RF2_18 (I/O), MSD_D3RF2_40 (I/O), MSD_D3RF2_48 (I/O), MSD_D3RF2_ODT150 (Input), MSD_D3RF2_ODT50 (Input), MSD_D3RF2_ODT75 (Input), MSD_D3RF2_ODTOFF (Input), MSD_D3RF3_34 (I/O), MSD_D3RF3_40 (I/O), MSD_D3RF3_48 (I/O), MSD_D3RF3L_34 (I/O), MSD_D3RF3L_40 (I/O), MSD_D3RF3L_48 (I/O), MSD_D3RF3L_ODT120 (Input), MSD_D3RF3L_ODT40 (Input), MSD_D3RF3L_ODT60 (Input), MSD_D3RF3L_ODTOFF (Input), MSD_D3RF3_ODT120 (Input), MSD_D3RF3_ODT40 (Input), MSD_D3RF3_ODT60 (Input), MSD_D3RF3_ODTOFF (Input)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
